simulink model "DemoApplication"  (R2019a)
settings: Solver=FixedStepDiscrete  StartTime=0.0  StopTime=0.01  FixedStep=m2c_ts  RelTol=1e-3  EnableMultiTasking=on
undefined symbols (not defined in the file): ModelParameter
libraries: General x12, Basic x3

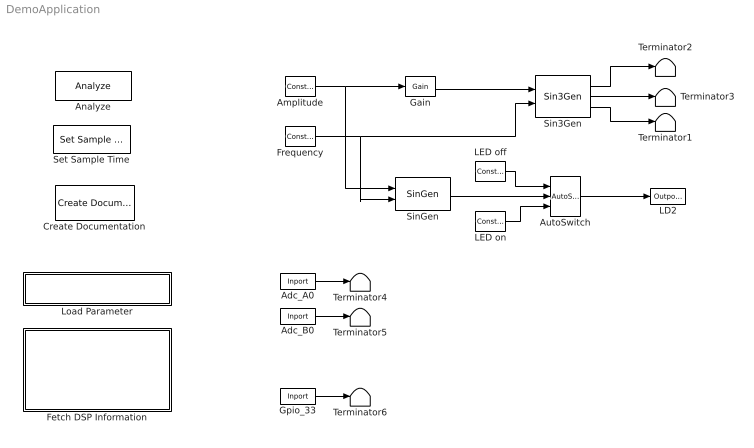
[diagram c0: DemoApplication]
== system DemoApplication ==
  Adc_A0 : General/Inport  DataType=int16  ts_fact=1.0  x2c_cfg_enableStaticId=off  x2c_cfg_staticId=0  BlockName=Inport  gain=1  offset=0
  Adc_B0 : General/Inport  DataType=int16  ts_fact=1.0  x2c_cfg_enableStaticId=off  x2c_cfg_staticId=0  BlockName=Inport  gain=1  offset=0
  Amplitude : General/Constant  Value=1  M2CAutoParam_UsedImplementation=16 Bit Fixed Point  x2c_cfg_enableStaticId=off  x2c_cfg_staticId=1  x2c_cfg_enableCot=off  BlockName=Constant
  Analyze : Basic/Analyze
  AutoSwitch : General/AutoSwitch  Thresh_up=0  Thresh_down=0  M2CAutoParam_UsedImplementation=16 Bit Fixed Point  x2c_cfg_enableStaticId=off  x2c_cfg_staticId=1  x2c_cfg_enableCot=off  BlockName=AutoSwitch
  Create Documentation : Basic/Create Documentation
  Fetch DSP Information : Subsystem
  Frequency : General/Constant  Value=2/1000  M2CAutoParam_UsedImplementation=16 Bit Fixed Point  x2c_cfg_enableStaticId=off  x2c_cfg_staticId=1  x2c_cfg_enableCot=off  BlockName=Constant
  Gain : General/Gain  Gain=0.2  M2CAutoParam_UsedImplementation=16 Bit Fixed Point  x2c_cfg_enableStaticId=off  x2c_cfg_staticId=1  x2c_cfg_enableCot=off  BlockName=Gain
  Gpio_33 : General/Inport  DataType=int16  ts_fact=1.0  x2c_cfg_enableStaticId=off  x2c_cfg_staticId=0  BlockName=Inport  gain=1  offset=0
  LD2 : General/Outport  DataType=int16  ts_fact=1.0  x2c_cfg_enableStaticId=off  x2c_cfg_staticId=0  BlockName=Outport  gain=1  offset=0
  LED off : General/Constant  Value=0.0  M2CAutoParam_UsedImplementation=16 Bit Fixed Point  x2c_cfg_enableStaticId=off  x2c_cfg_staticId=1  x2c_cfg_enableCot=off  BlockName=Constant
  LED on : General/Constant  Value=1  M2CAutoParam_UsedImplementation=16 Bit Fixed Point  x2c_cfg_enableStaticId=off  x2c_cfg_staticId=1  x2c_cfg_enableCot=off  BlockName=Constant
  Load Parameter : Subsystem  LoadFcn=ModelParameter;
  Set Sample Time : Basic/Set Sample Time  SampleTime=100e-6
  Sin3Gen : General/Sin3Gen  fmax=1000.0  ts_fact=1.0  M2CAutoParam_UsedImplementation=16 Bit Fixed Point  x2c_cfg_enableStaticId=off  x2c_cfg_staticId=1  x2c_cfg_enableCot=off  BlockName=Sin3Gen
  SinGen : General/SinGen  fmax=1000  Phase=0.0  ts_fact=1.0  M2CAutoParam_UsedImplementation=16 Bit Fixed Point  x2c_cfg_enableStaticId=off  x2c_cfg_staticId=1  x2c_cfg_enableCot=off  BlockName=SinGen
  Terminator{1..6} (6 alike) : Terminator
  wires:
  LED on/1 -> AutoSwitch/3
  AutoSwitch/1 -> LD2/1
  SinGen/1 -> AutoSwitch/2
  Frequency/1 -> Sin3Gen/2, SinGen/2
  Amplitude/1 -> SinGen/1, Gain/1
  Sin3Gen/1 -> Terminator2/1
  Sin3Gen/2 -> Terminator3/1
  Sin3Gen/3 -> Terminator1/1
  Gain/1 -> Sin3Gen/1
  Gpio_33/1 -> Terminator6/1
  Adc_B0/1 -> Terminator5/1
  Adc_A0/1 -> Terminator4/1
  LED off/1 -> AutoSwitch/1

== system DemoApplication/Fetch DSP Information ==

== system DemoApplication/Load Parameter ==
